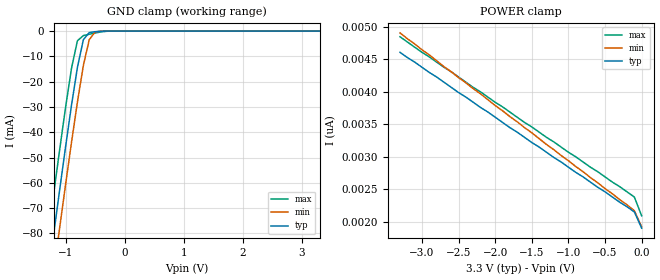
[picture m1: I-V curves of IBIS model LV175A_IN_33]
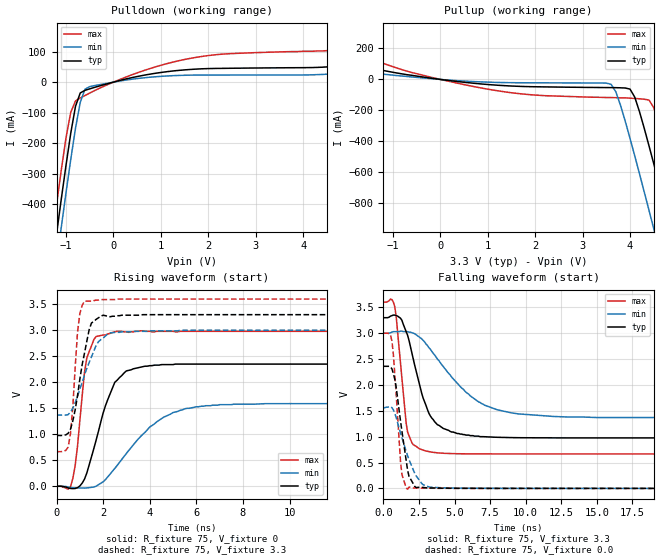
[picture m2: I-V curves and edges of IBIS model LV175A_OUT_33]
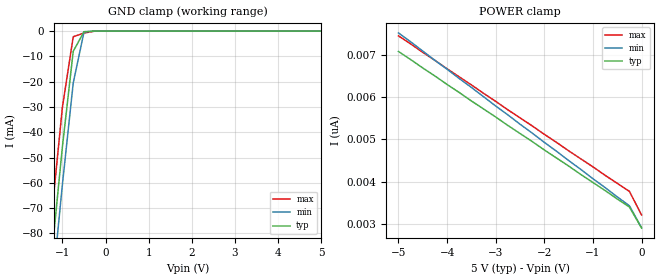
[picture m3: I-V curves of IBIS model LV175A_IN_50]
| TEXAS INSTRUMENTS INCORPORATED
| Standard Linear and Logic Group
| IBIS Model of SN74LV175A
| QUADRUPLE D-TYPE FLIP-FLOP WITH CLEAR
| SOIC 16-pin (D), SOP 16-pin (NS), SSOP 16-pin (DB), TSSOP 16-pin (PW)
| and TVSOP 16-pin (DGV) Package
[IBIS Ver]   3.2
[Comment Char]  |_char
[File Name]   lv175a.ibs
[File Rev]   2.0 H_die
[Date]   May 24, 2000
[Source]   Data created from HSPICE simulations at TI-SLL.
[Notes]   The following is an IBIS list for the LV175A.
|   Please contact sllibis@ti.com with questions and
|   comments concerning SLL IBIS models.
[Disclaimer] Property of Texas Instruments Incorporated.  Unauthorized
   reproduction and/or distribution is strictly prohibited.
   This product is protected under copyright law.
   Created 2000, (C) Copyright 2000, Texas Instruments Inc.,
   All Rights Reserved.
   UNLESS THERE IS A SIGNED, WRITTEN AGREEMENT TO THE
   CONTRARY, TEXAS INSTRUMENTS () IS PROVIDING THE IBIS
   MODELS  AND WITHOUT ANY WARRANTY, EXPRESSED OR
   IMPLIED.  TI assumes no liability for:
   1) the accuracy of the IBIS models provided to your
   company;
   2) the proper functioning of these IBIS Models in your
   design or for any resulting applications; or
   3) infringement of patents, copyrights or intellectual
   property rights resulting from your use of these IBIS
   models.
   TI provides IBIS Models as a service to our customers.
   You and your company shall not distribute, sell or give
   these models to anyone else without prior written
   permission from TI.
   TI reserves the right to make changes to our products or
   to discontinue any semiconductor product or service
   without notice, and advises our customers to obtain the
   latest version of relevant information to verify, before
   placing orders, that the information being relied on is
   current.
   Please be aware that your receipt and use of the IBIS
   information provided shall serve as acceptance of these
   terms and conditions.  If you do not accept these terms,
   you should return or destroy the IBIS models and any
   other accompanying information immediately.
|   Component LV175A_D
[Component]   LV175A_D
[Manufacturer]  Texas Instruments, Inc.
[Package]
|   typ   min   max
R_pkg   0.039   0.028   0.049
L_pkg   3.453nH   2.350nH   4.375nH
C_pkg   0.521pF   0.254pF   0.708pF
[Pin]   signal_name   model_name   R_pin   L_pin   C_pin
1   CLR_NOT   LV175A_IN   0.042   4.336nH   0.703pF
2   1Q   LV175A_OUT   0.049   3.778nH   0.634pF
3   1Q_NOT   LV175A_OUT   0.028   3.449nH   0.518pF
4   1D   LV175A_IN   0.029   2.393nH   0.254pF
5   2D   LV175A_IN   0.028   2.350nH   0.264pF
6   2Q_NOT   LV175A_OUT   0.048   3.312nH   0.483pF
7   2Q   LV175A_OUT   0.043   3.629nH   0.604pF
8   GND   GND   0.044   4.375nH   0.708pF
9   CLK   LV175A_IN   0.042   4.336nH   0.703pF
10   3Q   LV175A_OUT   0.049   3.778nH   0.634pF
11   3Q_NOT   LV175A_OUT   0.028   3.449nH   0.518pF
12   3D   LV175A_IN   0.029   2.393nH   0.255pF
13   4D   LV175A_IN   0.028   2.350nH   0.264pF
14   4Q_NOT   LV175A_OUT   0.048   3.312nH   0.483pF
15   4Q   LV175A_OUT   0.043   3.629nH   0.604pF
16   VCC   POWER   0.044   4.375nH   0.708pF
|   Component LV175A_NS
[Component]   LV175A_NS
[Manufacturer]  Texas Instruments, Inc.
[Package]
|   typ   min   max
R_pkg   0.042   0.035   0.049
L_pkg   3.147nH   2.164nH   4.219nH
C_pkg   0.404pF   0.241pF   0.562pF
[Pin]   signal_name   model_name   R_pin   L_pin   C_pin
1   CLR_NOT   LV175A_IN   0.049   4.215nH   0.562pF
2   1Q   LV175A_OUT   0.046   3.675nH   0.480pF
3   1Q_NOT   LV175A_OUT   0.037   2.527nH   0.332pF
4   1D   LV175A_IN   0.035   2.164nH   0.241pF
5   2D   LV175A_IN   0.035   2.164nH   0.241pF
6   2Q_NOT   LV175A_OUT   0.037   2.527nH   0.332pF
7   2Q   LV175A_OUT   0.046   3.675nH   0.480pF
8   GND   GND   0.049   4.215nH   0.562pF
9   CLK   LV175A_IN   0.049   4.219nH   0.562pF
10   3Q   LV175A_OUT   0.046   3.679nH   0.480pF
11   3Q_NOT   LV175A_OUT   0.037   2.531nH   0.333pF
12   3D   LV175A_IN   0.035   2.168nH   0.241pF
13   4D   LV175A_IN   0.035   2.168nH   0.241pF
14   4Q_NOT   LV175A_OUT   0.037   2.531nH   0.333pF
15   4Q   LV175A_OUT   0.046   3.679nH   0.480pF
16   VCC   POWER   0.049   4.219nH   0.562pF
|   Component LV175A_DB
[Component]   LV175A_DB
[Manufacturer]  Texas Instruments, Inc.
[Package]
|   typ   min   max
R_pkg   0.048   0.046   0.050
L_pkg   3.536nH   3.213nH   3.798nH
C_pkg   0.376pF   0.314pF   0.440pF
[Pin]   signal_name   model_name   R_pin   L_pin   C_pin
1   CLR_NOT   LV175A_IN   0.048   3.797nH   0.377pF
2   1Q   LV175A_OUT   0.046   3.723nH   0.440pF
3   1Q_NOT   LV175A_OUT   0.048   3.409nH   0.372pF
4   1D   LV175A_IN   0.049   3.213nH   0.314pF
5   2D   LV175A_IN   0.049   3.213nH   0.314pF
6   2Q_NOT   LV175A_OUT   0.048   3.409nH   0.372pF
7   2Q   LV175A_OUT   0.046   3.723nH   0.440pF
8   GND   GND   0.048   3.798nH   0.377pF
9   CLK   LV175A_IN   0.048   3.797nH   0.377pF
10   3Q   LV175A_OUT   0.046   3.725nH   0.440pF
11   3Q_NOT   LV175A_OUT   0.048   3.409nH   0.372pF
12   3D   LV175A_IN   0.049   3.214nH   0.314pF
13   4D   LV175A_IN   0.050   3.216nH   0.314pF
14   4Q_NOT   LV175A_OUT   0.048   3.409nH   0.372pF
15   4Q   LV175A_OUT   0.047   3.729nH   0.440pF
16   VCC   POWER   0.048   3.797nH   0.377pF
|   Component LV175A_PW
[Component]   LV175A_PW
[Manufacturer]  Texas Instruments, Inc.
[Package]
|   typ   min   max
R_pkg   0.045   0.038   0.051
L_pkg   2.593nH   2.447nH   3.080nH
C_pkg   0.281pF   0.243pF   0.377pF
[Pin]   signal_name   model_name   R_pin   L_pin   C_pin
1   CLR_NOT   LV175A_IN   0.040   3.080nH   0.377pF
2   1Q   LV175A_OUT   0.038   2.458nH   0.281pF
3   1Q_NOT   LV175A_OUT   0.051   2.512nH   0.255pF
4   1D   LV175A_IN   0.051   2.447nH   0.243pF
5   2D   LV175A_IN   0.051   2.447nH   0.243pF
6   2Q_NOT   LV175A_OUT   0.051   2.512nH   0.255pF
7   2Q   LV175A_OUT   0.038   2.458nH   0.281pF
8   GND   GND   0.040   3.080nH   0.377pF
9   CLK   LV175A_IN   0.039   2.832nH   0.316pF
10   3Q   LV175A_OUT   0.038   2.460nH   0.279pF
11   3Q_NOT   LV175A_OUT   0.051   2.512nH   0.255pF
12   3D   LV175A_IN   0.051   2.447nH   0.243pF
13   4D   LV175A_IN   0.051   2.447nH   0.243pF
14   4Q_NOT   LV175A_OUT   0.051   2.512nH   0.255pF
15   4Q   LV175A_OUT   0.038   2.459nH   0.279pF
16   VCC   POWER   0.039   2.832nH   0.316pF
|   Component LV175A_DGV
[Component]   LV175A_DGV
[Manufacturer]  Texas Instruments, Inc.
[Package]
|   typ   min   max
R_pkg   0.039   0.033   0.045
L_pkg   2.543nH   2.320nH   2.938nH
C_pkg   0.386pF   0.334pF   0.449pF
[Pin]   signal_name   model_name   R_pin   L_pin   C_pin
1   CLR_NOT   LV175A_IN   0.035   2.907nH   0.417pF
2   1Q   LV175A_OUT   0.042   2.558nH   0.446pF
3   1Q_NOT   LV175A_OUT   0.038   2.341nH   0.345pF
4   1D   LV175A_IN   0.038   2.320nH   0.334pF
5   2D   LV175A_IN   0.039   2.322nH   0.334pF
6   2Q_NOT   LV175A_OUT   0.038   2.353nH   0.342pF
7   2Q   LV175A_OUT   0.040   2.536nH   0.441pF
8   GND   GND   0.033   2.897nH   0.418pF
9   CLK   LV175A_IN   0.035   2.927nH   0.419pF
10   3Q   LV175A_OUT   0.045   2.632nH   0.449pF
11   3Q_NOT   LV175A_OUT   0.039   2.368nH   0.347pF
12   3D   LV175A_IN   0.039   2.330nH   0.335pF
13   4D   LV175A_IN   0.039   2.320nH   0.335pF
14   4Q_NOT   LV175A_OUT   0.039   2.361nH   0.345pF
15   4Q   LV175A_OUT   0.041   2.573nH   0.446pF
16   VCC   POWER   0.035   2.938nH   0.420pF
[Model Selector]   LV175A_IN
LV175A_IN_33   3.3-V Vcc Input Model
LV175A_IN_50   5.0-V Vcc Input Model
[Model Selector]   LV175A_OUT
LV175A_OUT_33   3.3-V Vcc Output Model
LV175A_OUT_50   5.0-V Vcc Output Model
| Models and submodels in the file (4): LV175A_IN_33 (Input), LV175A_OUT_33 (Output), LV175A_IN_50 (Input), LV175A_OUT_50 (Output)
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|   Model LV175A_IN_33
[Model]   LV175A_IN_33
Model_type  Input
Polarity   Inverting
Vinl = 0.99
Vinh = 2.31
| variable   typ   min   max
C_comp   1.43pf   1.07pf   1.79pf
[Temperature Range]   25   85   -40
[Voltage Range]   3.3   3.0   3.6
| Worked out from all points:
|   GND clamp passes 1 mA (typ) near -0.61 V on its own axis
[GND Clamp]
|   Voltage   I(typ)   I(min)   I(max)
-3.3V     -460mA     -475mA     -445mA
-1.3V     -97.5mA    -113mA     -81.5mA
-1.2V     -79.9mA    -95mA      -63.9mA
-1.1V     -62.6mA    -77.6mA    -46.7mA
-1V       -45.6mA    -60.5mA    -30mA
-900mV    -29.2mA    -43.9mA    -14.6mA
-800mV    -14.3mA    -28mA      -3.81mA
-700mV    -3.42mA    -13.6mA    -1.78mA
-600mV    -581uA     -3.4mA     -1.25mA
-500mV    -233uA     -353uA     -759uA
-400mV    -58.1uA    -21.9uA    -324uA
3.3V      1.9nA      2.34nA     1.69nA
[POWER Clamp]
|   Voltage   I(typ)   I(min)   I(max)
-3.3V     4.61nA     4.91nA     4.85nA
-3V       4.38nA     4.65nA     4.61nA
-100mV    2.15nA     2.17nA     2.38nA
0V        1.9nA      1.92nA     2.09nA
|   Model LV175A_OUT_33
[Model]   LV175A_OUT_33
Model_type  Output
Polarity   Non-Inverting
Vmeas = 1.65v
Cref = 15pf
| variable   typ   min   max
C_comp   4.62pf   3.47pf   5.77pf
[Temperature Range]   25   85   -40
[Voltage Range]   3.3   3.0   3.6
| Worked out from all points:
|   slope of the pulldown table from 0 to 0.495 V, typ, clamps not added: 27.3 ohm
|   slope of the pullup table from 0 to 0.495 V, typ, clamps not added: 27.2 ohm
|   rising waveform, R_fixture 75, V_fixture 0: 20-80 % time 954ps typ, 1.96ns min, 416ps max; typ from 0 V to 2.35 V
|   falling waveform, R_fixture 75, V_fixture 3.3: 20-80 % time 1.4ns typ, 3.23ns min, 602ps max; typ from 3.3 V to 0.976 V
|   rising waveform, R_fixture 75, V_fixture 3.3: 20-80 % time 534ps typ, 796ps min, 269ps max; typ from 0.976 V to 3.3 V
|   falling waveform, R_fixture 75, V_fixture 0.0: 20-80 % time 708ps typ, 1.15ns min, 433ps max; typ from 2.36 V to 0 V
[Pulldown]
|   Voltage   I(typ)   I(min)   I(max)
-3.3V     -3.04A     -3.13A     -2.95A
-1.3V     -615mA     -707mA     -518mA
-1.2V     -498mA     -591mA     -401mA
-1.1V     -383mA     -475mA     -288mA
-900mV    -167mA     -253mA     -98.6mA
-800mV    -79.1mA    -151mA     -61.7mA
-700mV    -35.5mA    -66.4mA    -51.9mA
-600mV    -26.8mA    -23.2mA    -43.9mA
-500mV    -22mA      -14.7mA    -35.8mA
1.6V      41.2mA     22.8mA     77.1mA
4.7V      52.3mA     27.8mA     106mA
6.6V      95.5mA     55.2mA     176mA
[Pullup]
|   Voltage   I(typ)   I(min)   I(max)
-3.3V     179mA      101mA      329mA
500mV     -18.4mA    -10.6mA    -33.4mA
3.6V      -52.9mA    -31.5mA    -117mA
3.8V      -54.2mA    -168mA     -119mA
4V        -62.6mA    -381mA     -121mA
4.1V      -115mA     -494mA     -123mA
4.4V      -429mA     -845mA     -133mA
4.5V      -544mA     -964mA     -182mA
4.8V      -899mA     -1.32A     -505mA
4.9V      -1.02A     -1.44A     -622mA
5.2V      -1.38A     -1.81A     -981mA
6.6V      -3.09A     -3.52A     -2.69A
[Ramp]
| variable   typ   min   max
dV/dt_r   1.42E+00/9.36E-10   9.69E-01/2.01E-09   1.80E+00/4.00E-10
dV/dt_f   1.43E+00/1.41E-09   1.00E+00/3.29E-09   1.80E+00/5.69E-10
R_load = 75
[Rising Waveform]
R_fixture = 75
V_fixture = 0
|   Time   V(typ)   V(min)   V(max)
0s        0V         0V         0V
500ps     -30.7mV    -12.3mV    -54.1mV
700ps     -43.6mV    -26.3mV    152mV
1.3ns     256mV      -30.4mV    2.47V
1.7ns     890mV      3.42mV     2.88V
2.5ns     2V         345mV      2.97V
3.8ns     2.31V      1.04V      2.98V
5ns       2.34V      1.42V      2.98V
7ns       2.35V      1.57V      2.98V
25ns      2.35V      1.59V      2.98V
[Falling Waveform]
R_fixture = 75
V_fixture = 3.3
V_fixture_min = 3.0
V_fixture_max = 3.6
|   Time   V(typ)   V(min)   V(max)
0s        3.3V       3V         3.6V
600ps     3.34V      3.02V      3.65V
800ps     3.35V      3.03V      3.51V
1.7ns     2.96V      3.03V      1.09V
2.5ns     2.05V      2.93V      771mV
3.2ns     1.45V      2.72V      712mV
3.8ns     1.23V      2.5V       687mV
6.1ns     1.02V      1.79V      668mV
8ns       988mV      1.52V      666mV
25ns      976mV      1.37V      666mV
[Rising Waveform]
R_fixture = 75
V_fixture = 3.3
V_fixture_min = 3.0
V_fixture_max = 3.6
|   Time   V(typ)   V(min)   V(max)
0s        976mV      1.37V      666mV
500ps     1.02V      1.38V      757mV
700ps     1.26V      1.5V       1.53V
900ps     1.74V      1.73V      2.96V
1ns       2.06V      1.87V      3.32V
1.2ns     2.56V      2.14V      3.56V
1.5ns     3.14V      2.49V      3.56V
1.8ns     3.24V      2.78V      3.58V
2.5ns     3.27V      2.96V      3.59V
25ns      3.3V       3V         3.6V
[Falling Waveform]
R_fixture = 75
V_fixture = 0.0
|   Time   V(typ)   V(min)   V(max)
0s        2.36V      1.56V      3V
400ps     2.36V      1.58V      2.99V
600ps     2.31V      1.56V      2.85V
900ps     1.95V      1.37V      1.81V
1.2ns     1.31V      1.07V      529mV
1.3ns     1.11V      981mV      272mV
1.7ns     353mV      631mV      -14.8mV
2.3ns     16.3mV     241mV      9.12mV
3.3ns     8.63mV     23.8mV     3.49mV
25ns      0V         0V         6.33uV
|   Model LV175A_IN_50
[Model]   LV175A_IN_50
Model_type  Input
Polarity   Inverting
Vinl = 1.5
Vinh = 3.5
| variable   typ   min   max
C_comp   1.43pf   1.07pf   1.79pf
[Temperature Range]   25   85   -40
[Voltage Range]   5.0   4.5   5.5
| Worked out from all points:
|   GND clamp passes 1 mA (typ) near -0.52 V on its own axis
[GND Clamp]
|   Voltage   I(typ)   I(min)   I(max)
-5V       -773mA     -786mA     -758mA
-1.5V     -133mA     -148mA     -117mA
-1.25V    -88.7mA    -104mA     -72.7mA
-1V       -45.6mA    -60.5mA    -30mA
-750mV    -7.99mA    -20.5mA    -2.23mA
-500mV    -233uA     -353uA     -759uA
-250mV    -2.63nA    -182nA     -26.9uA
5V        2.9nA      3.64nA     2.54nA
[POWER Clamp]
|   Voltage   I(typ)   I(min)   I(max)
-5V       7.08nA     7.52nA     7.45nA
-1.5V     4.37nA     4.5nA      4.73nA
-250mV    3.4nA      3.43nA     3.77nA
0V        2.9nA      2.91nA     3.21nA
